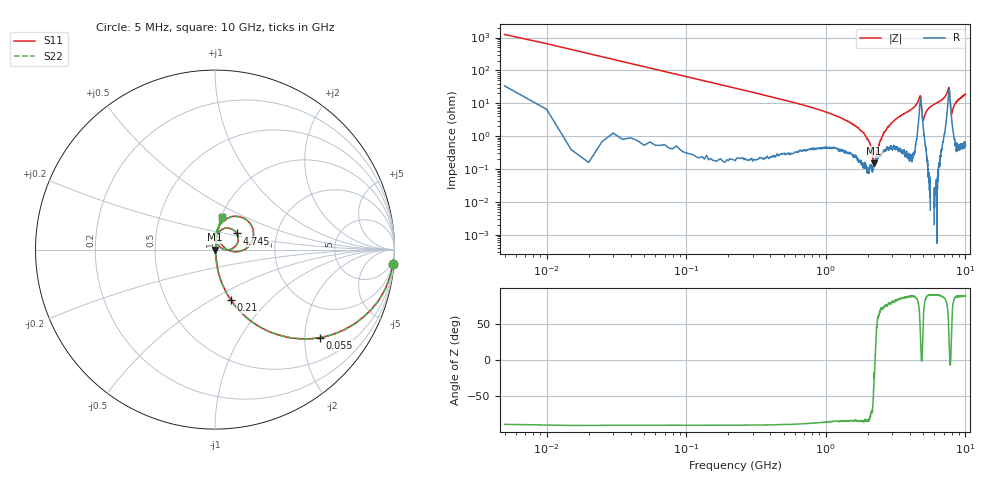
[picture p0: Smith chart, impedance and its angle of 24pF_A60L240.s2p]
! Amotech Co.,Ltd.
! http://www.amotech.co.kr/
! Part Number: A60L240
! These Parameters are Measured in Series Mode Connection
! Operation Temp=25[degC], DC Bias Voltage=0[V]
! Freq. Start=5[MHz] Stop=10[GHz], 2000[Steps]
! Date: Monday, July 14, 2020, 09:38:12
# GHZ S RI R 50.000000
!Freq.(Hz) S11(Real) S11(Imag) S21(Real) S21(Imag) S12(Real) S12(Imag) S22(Real) S22(Imag)
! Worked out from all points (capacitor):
!   2000 points, 5 MHz to 10 GHz, reference 50 ohm
!   read as one part in series: C = 24.3 pF near 55 MHz
!   lowest |Z| = 149 mohm at 2.215 GHz (marker M1)
!   series resonance near 2.256 GHz, so ESL is about 200 pH
!   S11 on the Smith chart (normalised r, x): 5 MHz: 2, -25; 55 MHz: 1.01, -2.38; 210 MHz: 1.00, -0.62; 4.745 GHz: 1.25, +0.23; 10 GHz: 1.01, +0.38
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0.005  0.9913 -0.08  0.00866 0.08  0.00866 0.08  0.9913 -0.08
0.055  0.5851 -0.4899  0.4149 0.4899  0.4149 0.4899  0.5851 -0.4899
0.12  0.2298 -0.4186  0.7702 0.4186  0.7702 0.4186  0.2298 -0.4186
0.21  0.0895 -0.2823  0.9105 0.2823  0.9105 0.2823  0.0895 -0.2823
0.57  0.0148 -0.1083  0.9852 0.1083  0.9852 0.1083  0.0148 -0.1083
1.675  0.00267 -0.0188  0.9973 0.0188  0.9973 0.0188  0.00267 -0.0188
2.045  0.000817 -0.00673  0.9992 0.00673  0.9992 0.00673  0.000817 -0.00673
2.215  0.00134 -0.000656  0.9987 0.000656  0.9987 0.000656  0.00134 -0.000656
2.43  0.00263 0.00588  0.9974 -0.00588  0.9974 -0.00588  0.00263 0.00588
2.61  0.00373 0.0123  0.9963 -0.0123  0.9963 -0.0123  0.00373 0.0123
3.34  0.00536 0.0382  0.9946 -0.0382  0.9946 -0.0382  0.00536 0.0382
4.24  0.00835 0.0721  0.9917 -0.0721  0.9917 -0.0721  0.00835 0.0721
4.745  0.1214 0.0898  0.8786 -0.0898  0.8786 -0.0898  0.1214 0.0898
4.93  0.0319 0.0106  0.9681 -0.0106  0.9681 -0.0106  0.0319 0.0106
5.005  0.0164 0.0266  0.9836 -0.0266  0.9836 -0.0266  0.0164 0.0266
5.485  0.00583 0.0719  0.9942 -0.0719  0.9942 -0.0719  0.00583 0.0719
6.67  0.0172 0.1187  0.9828 -0.1187  0.9828 -0.1187  0.0172 0.1187
7.58  0.1954 0.1463  0.8046 -0.1463  0.8046 -0.1463  0.1954 0.1463
7.685  0.1927 0.0241  0.8073 -0.0241  0.8073 -0.0241  0.1927 0.0241
7.94  0.0384 0.0253  0.9616 -0.0253  0.9616 -0.0253  0.0384 0.0253
8.335  0.0153 0.0853  0.9847 -0.0853  0.9847 -0.0853  0.0153 0.0853
10  0.0398 0.1822  0.9602 -0.1822  0.9602 -0.1822  0.0398 0.1822
